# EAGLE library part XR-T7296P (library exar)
DS3/Sonet STS-1 LINE DRIVER
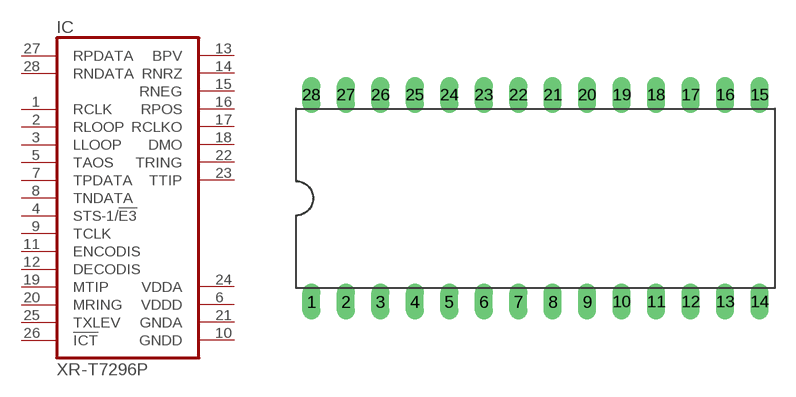
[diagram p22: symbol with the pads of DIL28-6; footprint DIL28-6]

Designator prefix IC

## XR-T7296P (OC_FARNELL: unknown; OC_NEWARK: unknown)  [DIL28-6]
1  RCLK  in
2  RLOOP  in
3  LLOOP  in
4  STS-1/!E3  in
5  TAOS  in
6  VDDD  pwr
7  TPDATA  in
8  TNDATA  in
9  TCLK  in
10  GNDD  pwr
11  ENCODIS  in
12  DECODIS  in
13  BPV  out
14  RNRZ  out
15  RNEG  out
16  RPOS  out
17  RCLKO  out
18  DMO  out
19  MTIP  in
20  MRING  in
21  GNDA  pwr
22  TRING  out
23  TTIP  out
24  VDDA  pwr
25  TXLEV  in
26  !ICT  in
27  RPDATA  in
28  RNDATA  in

## Footprint DIL28-6 (pad centres in mm)
Dual In Line Package 0.6 inch
drill 0.813 long: 1 -16.51,-7.62; 2 -13.97,-7.62; 3 -11.43,-7.62; 4 -8.89,-7.62; 5 -6.35,-7.62; 6 -3.81,-7.62; 7 -1.27,-7.62; 8 1.27,-7.62; 9 3.81,-7.62; 10 6.35,-7.62; 11 8.89,-7.62; 12 11.43,-7.62; 13 13.97,-7.62; 14 16.51,-7.62; 15 16.51,7.62; 16 13.97,7.62; 17 11.43,7.62; 18 8.89,7.62; 19 6.35,7.62; 20 3.81,7.62; 21 1.27,7.62; 22 -1.27,7.62; 23 -3.81,7.62; 24 -6.35,7.62; 25 -8.89,7.62; 26 -11.43,7.62; 27 -13.97,7.62; 28 -16.51,7.62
